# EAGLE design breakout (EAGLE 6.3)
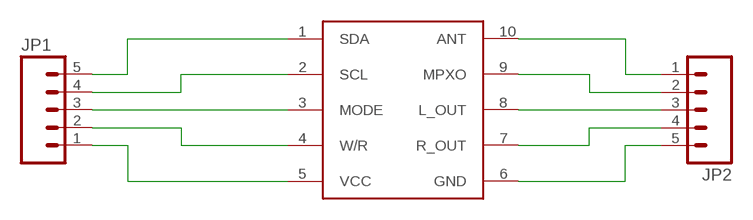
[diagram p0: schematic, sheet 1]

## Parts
JP1  M05LOCK_LONGPADS  [1X05_LOCK_LONGPADS]
JP2  M05LOCK_LONGPADS  [1X05_LOCK_LONGPADS]
U$1  TEA5767BREAKOUT  [TEA5767MM2]

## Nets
N$1: JP1.5 U$1.1(SDA)
N$2: JP1.4 U$1.2(SCL)
N$3: JP1.3 U$1.3(MODE)
N$4: JP1.2 U$1.4(W/R)
N$5: JP1.1 U$1.5(VCC)
N$6: JP2.1 U$1.10(ANT)
N$7: JP2.2 U$1.9(MPXO)
N$8: JP2.3 U$1.8(L_OUT)
N$9: JP2.4 U$1.7(R_OUT)
N$10: JP2.5 U$1.6(GND)

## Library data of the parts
JP1 JP2 = SparkFun-Connectors:M05: Header 5 Standard 5-pin 0.1" header. Use with straight break away headers (SKU : PRT-00116), right angle break away headers (PRT-00553), swiss pins (PRT-00743), machine pins (PRT-00117), and female headers (PRT-00115). Molex polarized connector foot print use with SKU : PRT-08230 with associated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
U$1 = MyParts:TEA5767BREAKOUT

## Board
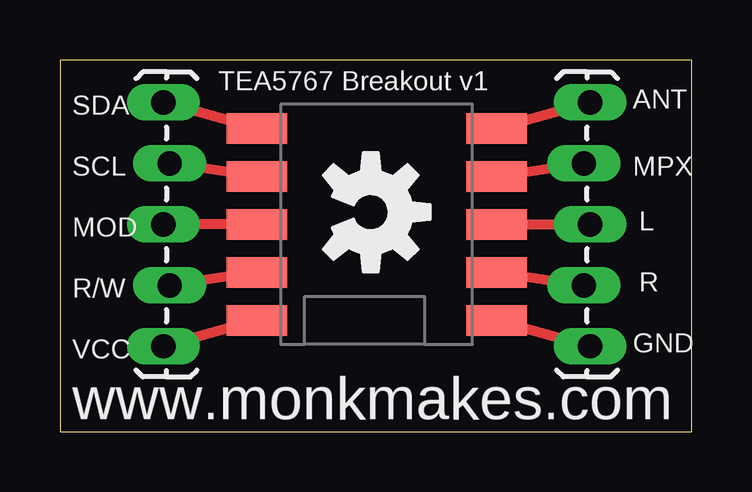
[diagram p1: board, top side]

Size 26.34 x 15.48 mm. Coordinates in mm from the lower left corner, seen from the top.
Outline: 0,0 26.34,0 26.34,15.48 0,15.48 0,0
Copper layers (1*16): Top 0.035mm / dielectric 1.5mm / Bottom 0.035mm
Design rules "default": minimum track width 10mil, minimum drill 24mil, track to track 8mil, track to pad 8mil, pad to pad 8mil, via to via 8mil, smd to smd 8mil, copper to edge 40mil, drill to drill 8mil, minimum pad ring 10mil, minimum via ring 8mil, stop-mask expansion 4mil, vias tented up to drill 0mil, thermal gap 10mil

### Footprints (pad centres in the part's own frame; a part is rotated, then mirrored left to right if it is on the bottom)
1X05_LOCK_LONGPADS = drill 1.016 long: 1 0,0; 2 2.54,-0.254; 3 5.08,0; 4 7.62,-0.254; 5 10.16,0
TEA5767MM2 = smd 2.54 x 1.27: 1 -5,4; 2 -5,2; 3 -5,0; 4 -5,-2; 5 -5,-4; 6 5,-4; 7 5,-2; 8 5,0; 9 5,2; 10 5,4

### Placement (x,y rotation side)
JP1  4.32,3.56 90 top
JP2  22.1,13.72 270 top
U$1  13.21,8.64 0 top
U$2  [OSHW-LOGO-M]  12.95,9.14 270 top

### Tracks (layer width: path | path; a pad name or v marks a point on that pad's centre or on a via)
N$1
  Top 0.406: U$1.1 JP1.5
N$2
  Top 0.406: U$1.2 JP1.4
N$3
  Top 0.406: U$1.3 JP1.3
N$4
  Top 0.406: U$1.4 JP1.2
N$5
  Top 0.406: U$1.5 JP1.1
N$6
  Top 0.406: U$1.10 JP2.1
N$7
  Top 0.406: U$1.9 JP2.2
N$8
  Top 0.406: U$1.8 JP2.3
N$9
  Top 0.406: U$1.7 JP2.4
N$10
  Top 0.406: U$1.6 JP2.5

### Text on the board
tPlace: TEA5767 Breakout v1 | ANT | SDA | SCL | MPX | L | MOD | R/W | R | GND | VCC | www.monkmakes.com

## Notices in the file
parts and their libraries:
SparkFun-Connectors: Licensing: CC v3.0 Share-Alike You are welcome to use this library for commercial purposes.
